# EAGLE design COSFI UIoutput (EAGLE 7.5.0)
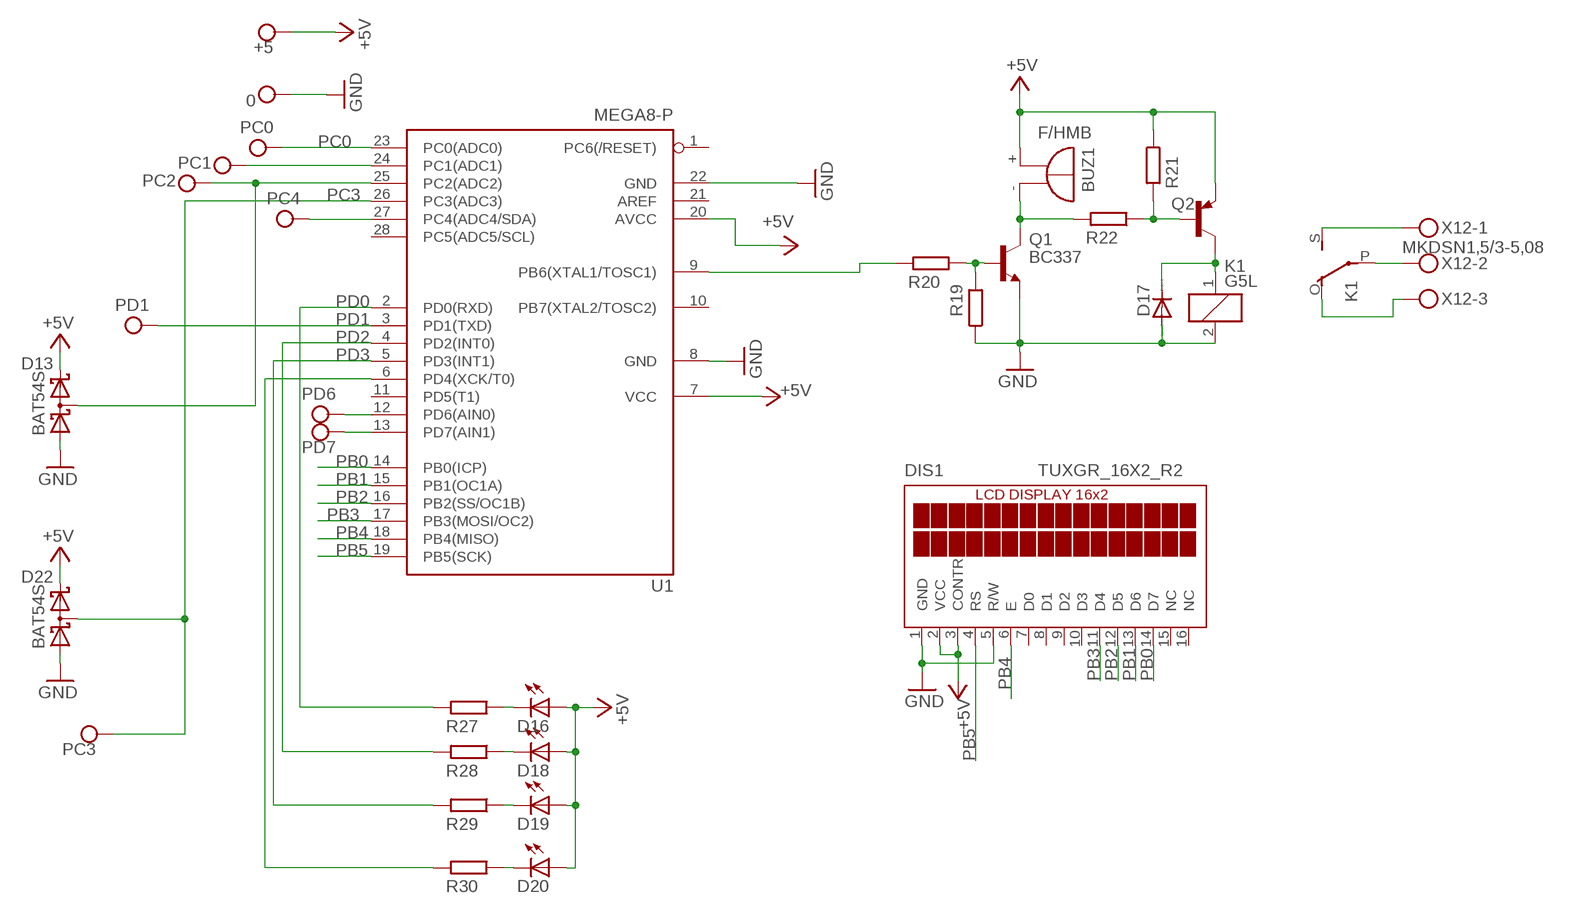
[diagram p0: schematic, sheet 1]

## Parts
0  CONNWIRE  [CONNWIRE]
+5  CONNWIRE  [CONNWIRE]
BUZ1  F/HMB  [F/HMB]
D13  BAT54S  [SOT23]
D16  LED3MM  [LED3MM]
D17  1N4004  [DO41-10]
D18  LED3MM  [LED3MM]
D19  LED3MM  [LED3MM]
D20  LED3MM  [LED3MM]
D22  BAT54S  [SOT23]
DIS1  TUXGR_16X2_R2  [TUXGR_16X2_R2]
K1  G5L  [G5LE]
PC0  CONNWIRE  [CONNWIRE]
PC1  CONNWIRE  [CONNWIRE]
PC2  CONNWIRE  [CONNWIRE]
PC3  CONNWIRE  [CONNWIRE]
PC4  CONNWIRE  [CONNWIRE]
PD1  CONNWIRE  [CONNWIRE]
PD6  CONNWIRE  [CONNWIRE]
PD7  CONNWIRE  [CONNWIRE]
Q1  BC337  [TO92]
Q2  -PNP-TO126  [TO126]
R19  R-EU_0204/7  [0204/7]
R20  R-EU_0204/7  [0204/7]
R21  R-EU_0204/7  [0204/7]
R22  R-EU_0204/7  [0204/7]
R27  R-EU_0204/7  [0204/7]
R28  R-EU_0204/7  [0204/7]
R29  R-EU_0204/7  [0204/7]
R30  R-EU_0204/7  [0204/7]
U1  MEGA8-P  [DIL28-3]
X12  MKDSN1,5/3-5,08  [MKDSN1,5/3-5,08]

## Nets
+5V: +5.P$1 BUZ1.+ D13.2(C2) D16.A D18.A D19.A D20.A D22.2(C2) DIS1.2(VCC) DIS1.3(CONTR) Q2.1(E) R21.1 U1.7(VCC) U1.20(AVCC)
GND: 0.P$1 D13.1(A1) D17.A D22.1(A1) DIS1.1(GND) DIS1.5(R/W) K1.2 Q1.1(E) R19.1 U1.8(GND) U1.22(GND)
N$1: PC1.P$1 U1.24(PC1(ADC1))
N$2: PD7.P$1 U1.13(PD7(AIN1))
N$4: D13.3(C1A2) PC2.P$1 U1.25(PC2(ADC2))
N$6: D16.K(C) R27.1
N$7: Q1.2(B) R19.2 R20.1
N$8: D18.K(C) R28.1
N$9: D19.K(C) R29.1
N$10: D20.K(C) R30.1
N$11: PC4.P$1 U1.27(PC4(ADC4/SDA))
N$12: PD6.P$1 U1.12(PD6(AIN0))
N$23: BUZ1.- Q1.3(C) R22.2
N$25: Q2.3(B) R21.2 R22.1
N$26: D17.C K1.1 Q2.2(C)
N$27: K1.P(2:P) X12.2
N$28: K1.O(2:O) X12.3
N$29: K1.S(2:S) X12.1
N$30: R20.2 U1.9(PB6(XTAL1/TOSC1))
PB0: DIS1.14(D7) U1.14(PB0(ICP))
PB1: DIS1.13(D6) U1.15(PB1(OC1A))
PB2: DIS1.12(D5) U1.16(PB2(SS/OC1B))
PB3: DIS1.11(D4) U1.17(PB3(MOSI/OC2))
PB4: DIS1.6(E) U1.18(PB4(MISO))
PB5: DIS1.4(RS) U1.19(PB5(SCK))
PC0: PC0.P$1 U1.23(PC0(ADC0))
PC3: D22.3(C1A2) PC3.P$1 U1.26(PC3(ADC3))
PD0: R27.2 U1.2(PD0(RXD))
PD1: PD1.P$1 R28.2 U1.3(PD1(TXD)) U1.4(PD2(INT0))
PD2: R29.2 U1.5(PD3(INT1))
PD3: R30.2 U1.6(PD4(XCK/T0))
Unconnected: DIS1.7(D0) DIS1.8(D1) DIS1.9(D2) DIS1.10(D3) DIS1.15(NC) DIS1.16(NC) U1.1(PC6(/RESET)) U1.10(PB7(XTAL2/TOSC2)) U1.11(PD5(T1)) U1.21(AREF) U1.28(PC5(ADC5/SCL))

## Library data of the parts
0 +5 PC0 PC1-PC4 PD1 PD6 PD7 = connholes:CONNWIRE
BUZ1 = buzzer:F/HMB: BUZZER; OC_FARNELL: unknown; OC_NEWARK: unknown
D13 D22 = diode:BAT54S: Schottky Diodes Pin connection corrected 2011-05-04 Source: Fairchild .. BAT54.pdf
D16 D18-D20 = led:LED: LED
D17 = diode:1N4004: DIODE
DIS1 = display-lcd:TUXGR_16X2_R2: Tuxgraphics LCD display 16x2 characters reflective, without background light Source: tuxgr_12x2_r2.pdf; OC_FARNELL: unknown; OC_NEWARK: unknown
K1 = relay:G5L: RELAY 1 x switch, 10 A/120 V AC, 8 A/30 V ADC, Omron; OC_FARNELL: unknown; OC_NEWARK: unknown
Q1 = transistor:BC337: NPN TRANSISTOR
Q2 = transistor:*-PNP-: PNP Transistror
R19-R22 R27-R30 = rcl:R-EU_: RESISTOR, European symbol
U1 = atmel:MEGA8-P: MICROCONTROLLER 8 Kbytes FLASH, 1 kbytes SRAM, 512 bytes EEPROM, USART, 4-channel 10 bit ADC, 2-channel 8 bit ADC Pin compatible with Atmega48, ATMega88, ATMega168 Source: avr.lbr; OC_FARNELL: unknown; OC_NEWARK: unknown
X12 = con-phoenix-508:MKDSN1,5/3-5,08: MKDSN 1,5/ 3-5,08 Printklemme Nennstrom: 13,5 A Nennspannung: 250 V Rastermaß: 5,08 mm Polzahl: 3 Anschlussart: Schraubanschluss Montage: Löten Anschlussrichtung Leiter/Platine: 0 ° Artikelnummer: 1729131 Source: http://eshop.phoenixcontact.com .. 1729131.pdf

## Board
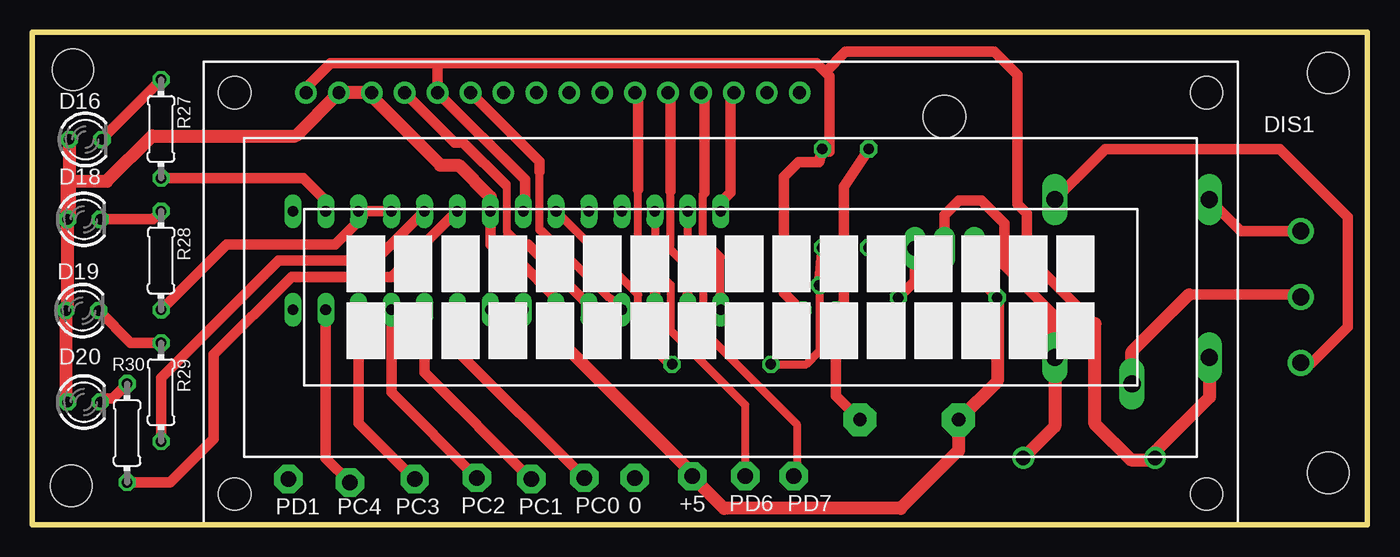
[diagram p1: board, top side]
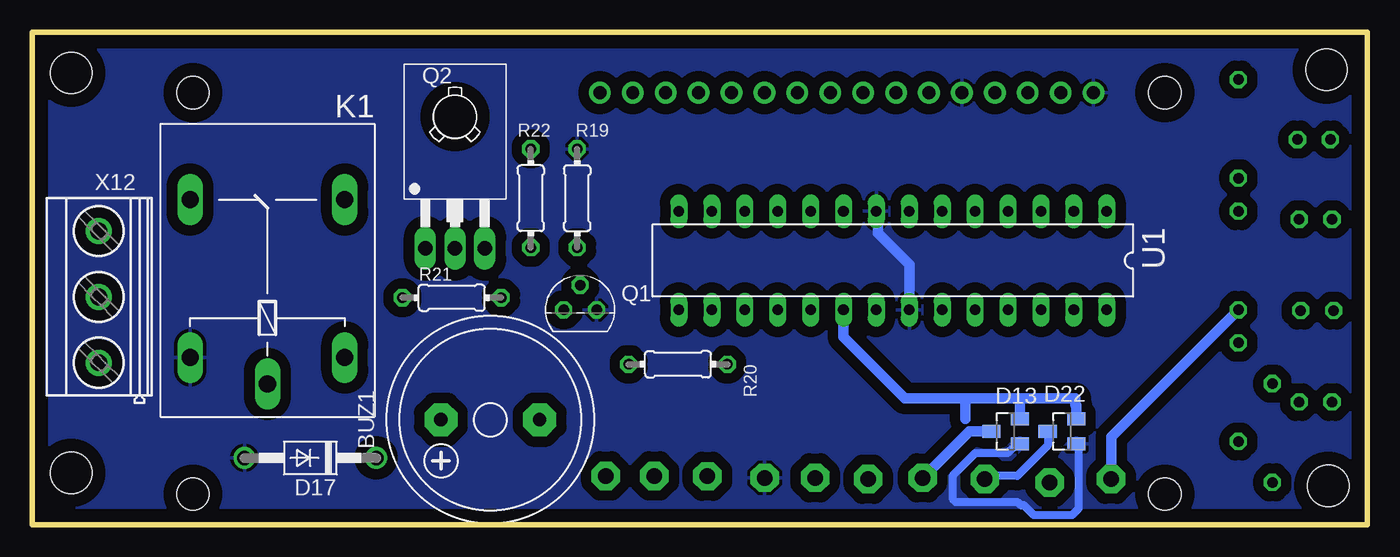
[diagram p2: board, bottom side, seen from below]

Size 103 x 38 mm. Coordinates in mm from the lower left corner, seen from the top.
Outline: 0,0 103,0 103,38 0,38 0,0
Copper layers (1*16): Top 0.035mm / dielectric 1.5mm / Bottom 0.035mm
Design rules "default": minimum track width 10mil, minimum drill 24mil, track to track 8mil, track to pad 8mil, pad to pad 8mil, via to via 8mil, smd to smd 8mil, copper to edge 40mil, drill to drill 8mil, minimum pad ring 10mil, minimum via ring 8mil, stop-mask expansion 4mil, vias tented up to drill 0mil, thermal gap 10mil
Holes 3.2 mm at 3,3 3.12,35.12 100,34.88 100,4

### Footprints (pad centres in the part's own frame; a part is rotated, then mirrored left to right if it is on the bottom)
CONNWIRE = drill 1.2 pad 2.184 octagon: P$1 0,0
F/HMB = drill 1.016 pad 2.54 octagon: + 3.81,0; - -3.81,0
SOT23 = smd 1 x 1.4: 1 -0.95,-1.1; 2 0.95,-1.1; 3 0,1.1
LED3MM = drill 0.813 octagon: A -1.27,0; K 1.27,0
DO41-10 = drill 1.118: A 5.08,0; C -5.08,0
TUXGR_16X2_R2 = drill 1 pad 1.676: 1 -32,15.5; 2 -29.46,15.5; 3 -26.92,15.5; 4 -24.38,15.5; 5 -21.84,15.5; 6 -19.3,15.5; 7 -16.76,15.5; 8 -14.22,15.5; 9 -11.68,15.5; 10 -9.14,15.5; 11 -6.6,15.5; 12 -4.06,15.5; 13 -1.52,15.5; 14 1.02,15.5; 15 3.56,15.5; 16 6.1,15.5 | hole 2.5: -37.5,-15.5; 37.5,-15.5; -37.5,15.5; 37.5,15.5
G5LE = drill 1.321 long: 1 -7.493,-5.969; 2 -7.493,5.969; O 4.699,5.969; P -9.525,0; S 4.699,-5.969
TO92 = drill 0.813 octagon: 1 1.27,0; 2 0,1.905; 3 -1.27,0
TO126 = drill 1.118 long: 1 -2.286,-5.08; 2 0,-5.08; 3 2.286,-5.08 | hole 3.302: 0,5.08
0204/7 = drill 0.813 octagon: 1 -3.81,0; 2 3.81,0
DIL28-3 = drill 0.813 long: 1 -16.51,-3.81; 2 -13.97,-3.81; 3 -11.43,-3.81; 4 -8.89,-3.81; 5 -6.35,-3.81; 6 -3.81,-3.81; 7 -1.27,-3.81; 8 1.27,-3.81; 9 3.81,-3.81; 10 6.35,-3.81; 11 8.89,-3.81; 12 11.43,-3.81; 13 13.97,-3.81; 14 16.51,-3.81; 15 16.51,3.81; 16 13.97,3.81; 17 11.43,3.81; 18 8.89,3.81; 19 6.35,3.81; 20 3.81,3.81; 21 1.27,3.81; 22 -1.27,3.81; 23 -3.81,3.81; 24 -6.35,3.81; 25 -8.89,3.81; 26 -11.43,3.81; 27 -13.97,3.81; 28 -16.51,3.81
MKDSN1,5/3-5,08 = drill 1.3 pad 2: 1 -7.641,0.025; 2 -2.561,0.025; 3 2.519,0.025

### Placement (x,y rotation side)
0  46.49,3.6 0 top
+5  50.91,3.73 0 top
BUZ1  67.67,8.1 180 bottom
D13  27.9,7.2 90 bottom
D16  4.1,29.73 0 top
D17  81.55,5.14 180 bottom
D18  3.98,23.57 0 top
D19  3.85,16.52 0 top
D20  3.98,9.46 0 top
D22  23.55,7.2 90 bottom
DIS1  53.11,17.84 0 top
K1  84.86,20.39 90 bottom
PC0  42.6,3.6 0 top
PC1  38.5,3.5 0 top
PC2  34.3,3.6 0 top
PC3  29.5,3.5 0 top
PC4  24.5,3.25 0 top
PD1  19.75,3.5 0 top
PD6  55,3.75 0 top
PD7  58.75,3.75 0 top
Q1  60.73,16.57 0 bottom
Q2  70.39,26.41 0 bottom
R19  60.96,25.2 270 bottom
R20  53.18,12.38 0 bottom
R21  70.64,17.52 0 bottom
R22  64.54,25.2 90 bottom
R27  9.93,30.55 270 top
R28  9.93,20.39 270 top
R29  9.93,10.22 270 top
R30  7.3,7.07 270 top
U1  36.6,20.39 180 bottom
X12  97.85,20.14 90 bottom

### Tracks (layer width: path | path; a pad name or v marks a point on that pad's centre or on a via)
+5V
  Top 0.813: U1.20 40.41,17.46 37.5,20.38 36.62,20.38 35.38,21.62 35.38,24.15 U1.7 | Q2.1 72.68,19.29 R21.1
  Top 1.016: U1.7 35.33,25.3 32.88,27.75 31.5,27.75 26.19,33.06 DIS1.3 DIS1.2 20.3,30 9.25,30 5.75,26.5 2.75,26.5 2.71,26.45 D18.A | D16.A 2.83,23.7 D18.A | D18.A 2.71,16.64 D19.A 2.58,9.59 D20.A | R21.1 74.45,11.07 BUZ1.+ 71.47,5.72 67,1.25 53.38,1.25 +5.P$1 50.91,4 40.41,14.5 U1.20
  Bottom 0.813: D22.2 22.45,9.2 22.5,9.25 22.5,9.75 26.75,9.75 | 26.75,9.75 31,9.75 | 31,9.75 31,8.17 | D13.2 26.8,9.7 26.75,9.75 | 31,9.75 35.66,9.75 40.41,14.5 U1.20
GND
  Top 0.813: DIS1.1 21.11,33.73 23,35.62 31,35.62 | U1.8 38,24.32 38,26.62 DIS1.5 31.27,35.35 31,35.62 | 61.19,34.94 61.5,34.62 61.5,28.8 R19.1 60.7,28 59.12,28 58,26.88 58,17.88 59.3,16.57 Q1.1 59.2,16.57 | 61.19,34.94 60.5,35.62 31,35.62 | 82,15.5 76.75,20.75 76.75,24 76,24.75 76,34.75 74.25,36.5 62.75,36.5 61.19,34.94
  Top 1.016: 82,15.5 82,7.75 84.75,5 86,5 | 86,5 86.48,5 D17.A | K1.2 90.83,9.83 86,5
  Bottom 0.61: D13.1 27,6.25 27.75,5.5 30.25,5.5 32,3.75 32,2 31.75,1.75 27,1.75 26.75,1.5 26.5,1.5 25.75,0.75 22.75,0.75 22.25,1.25 22.25,6.04 D22.1
  Bottom 0.813: U1.22 35.33,20.08 37.75,22.5 37.75,24.07 U1.8
  pour Bottom (isolate 0.813): 0.25,37.25 102.5,37.25 102.5,0.5 0.25,0.5
N$1
  Top 0.813: U1.24 30.25,11.75 PC1.P$1
N$2
  Top 0.61: U1.13 50.57,21.75 51.75,20.57 51.75,15 59,7.75 59,4 PD7.P$1
N$4
  Top 0.813: U1.25 27.71,10.19 PC2.P$1
  Bottom 0.813: D13.3 30.7,7.2 PC2.P$1
N$6
  Top 0.813: D16.K 5.37,29.8 R27.1
N$7
  Top 0.61: Q1.2 60.73,13.38 59.72,12.38 R20.1
  Top 0.813: R19.2 60.71,18.5 Q1.2
N$8
  Top 0.813: D18.K 9.3,23.57 R28.1
N$9
  Top 0.813: R29.1 7.6,14.04 D19.K
N$10
  Top 0.813: D20.K 5.25,9.49 5.5,9.75 6.18,9.75 R30.1
N$11
  Top 0.813: U1.27 22.63,5.12 PC4.P$1
N$12
  Top 0.61: U1.12 48.03,19.72 49.25,18.5 49.25,15 55,9.25 PD6.P$1
N$23
  Top 0.813: R22.2 62.62,26.09 62.62,17.2 Q1.3 62,9.95 BUZ1.-
N$25
  Top 0.813: R21.2 68.1,18.79 Q2.3 64.6,21.32 R22.1
N$26
  Top 0.813: Q2.2 70.39,23.89 71.5,25 73.25,25 75,23.25 75,20 78.75,16.25 78.75,13.03 K1.1
  Top 1.016: K1.1 78.89,7.57 D17.C
N$27
  Top 0.813: 89.25,17.75 97.88,17.75 X12.2
  Top 1.016: K1.P 84.86,13.36 89.25,17.75
N$28
  Top 0.813: X12.3 93.26,22.65 K1.O
N$29
  Top 0.813: X12.1 98.74,12.49 101.5,15.25 101.5,23.75 96.25,29 82.81,29 K1.S
N$30
  Top 0.61: 46.88,14.75 46.88,14.88 46.75,15 46.75,17.75 45.12,19.38 45.12,19.48 U1.9
  Top 0.813: R20.2 49.25,12.38 46.88,14.75
PB0
  Top 0.813: U1.14 53.11,24.86 53.88,25.62 53.88,33.09 DIS1.14
PB1
  Top 0.61: 53.11,17.64 53.11,20.64 51.75,22 51.75,25.5 51.88,25.62
  Top 0.813: U1.15 53.11,17.64 | 51.88,25.62 51.88,33.06 DIS1.13
PB2
  Top 0.61: 49.25,25.75 49.25,21.25 50.57,19.93 50.57,17.68
  Top 0.813: U1.16 50.57,17.68 | 49.25,25.75 49.25,33.15 DIS1.12
PB3
  Top 0.61: 46.75,19.38 46.75,25.88
  Top 0.813: U1.17 48.03,18.09 46.75,19.38 | 46.75,25.88 46.75,33.1 DIS1.11
PB4
  Top 0.406: 39.25,22.62 39.38,22.62 | 44.5,17.5 44.56,17.5
  Top 0.61: 39.25,22.62 39.12,22.75 39.12,27.25 | 39.38,22.62 44.5,17.5 | 44.56,17.5 U1.18
  Top 0.813: 39.12,27.25 39.12,28.03 DIS1.6
PB5
  Top 0.61: 36.75,22.38 36.75,22.5 36.62,22.62 36.62,26.12 36.5,26.25
  Top 0.813: 36.75,22.38 37.5,21.62 38.25,21.62 42.95,16.93 U1.19 | 36.5,26.25 33.25,29.5 32.58,29.5 DIS1.4
PC0
  Top 0.813: U1.23 32.79,13.41 PC0.P$1
PC3
  Top 0.813: U1.26 25.17,7.83 PC3.P$1
  Bottom 0.61: D22.3 24.65,6.1 27,3.75 29.25,3.75 PC3.P$1
PD0
  Top 0.813: R27.2 20.89,26.73 22.5,25.12 22.5,24.32 U1.2
PD1
  Top 0.813: R28.2 14.98,21.62 23.38,21.62 25.5,23.75 25.5,23.86 U1.3 U1.4
  Bottom 0.813: PD1.P$1 19.75,6.75 R28.2
PD2
  Top 0.813: R29.2 9.93,11.3 19,20.38 26.43,20.38 U1.5
PD3
  Top 0.813: R30.2 10.63,3.25 14,6.62 14,13.12 20,19.12 27.72,19.12 U1.6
